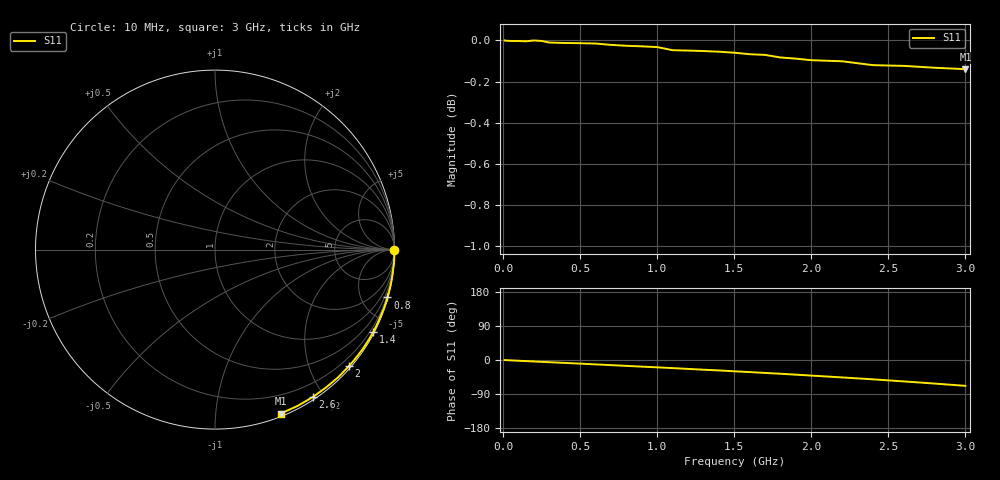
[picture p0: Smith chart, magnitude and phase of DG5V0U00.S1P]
! SIEMENS Small Signal Semiconductors
! BAV70
! Silicon Switching Diode in SOT23
! VR = 5 V
! S-Parameters:  May  1995
# GHz  S  MA  R  50
!  f  S11
! GHz  MAG  ANG
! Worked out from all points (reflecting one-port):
!   30 points, 10 MHz to 3 GHz, reference 50 ohm
!   lowest |S11| = -0.1 dB at 3 GHz (marker M1), VSWR 124.47, Z = 1.28 - j73.8 ohm
!   phase of S11 starts at -0 deg and turns -68 deg over the sweep
!   S11 on the Smith chart (normalised r, x): 10 MHz: open; 800 MHz: 0.08, -7.35; 1.4 GHz: 0.06, -4.09; 2 GHz: 0.04, -2.67; 2.6 GHz: 0.03, -1.86; 3 GHz: 0.03, -1.48
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0.01  1 -0.2
0.1  0.9997 -2.0
0.15  0.9995 -2.9
0.2  1 -3.9
0.25  0.9997 -4.9
0.3  0.9988 -5.8
0.4  0.9986 -7.7
0.5  0.9985 -9.6
0.6  0.9983 -11.6
0.7  0.9975 -13.5
0.8  0.997 -15.5
0.9  0.9967 -17.5
1  0.9963 -19.4
1.1  0.9946 -21.4
1.2  0.9943 -23.5
1.3  0.9941 -25.6
1.4  0.9937 -27.5
1.5  0.9932 -29.8
1.6  0.9923 -31.9
1.7  0.9919 -34.1
1.8  0.9905 -36.3
1.9  0.9899 -38.7
2  0.989 -41.1
2.2  0.9884 -46.0
2.4  0.9863 -51.0
2.6  0.9859 -56.5
2.8  0.9848 -62.2
3  0.9841 -68.2
